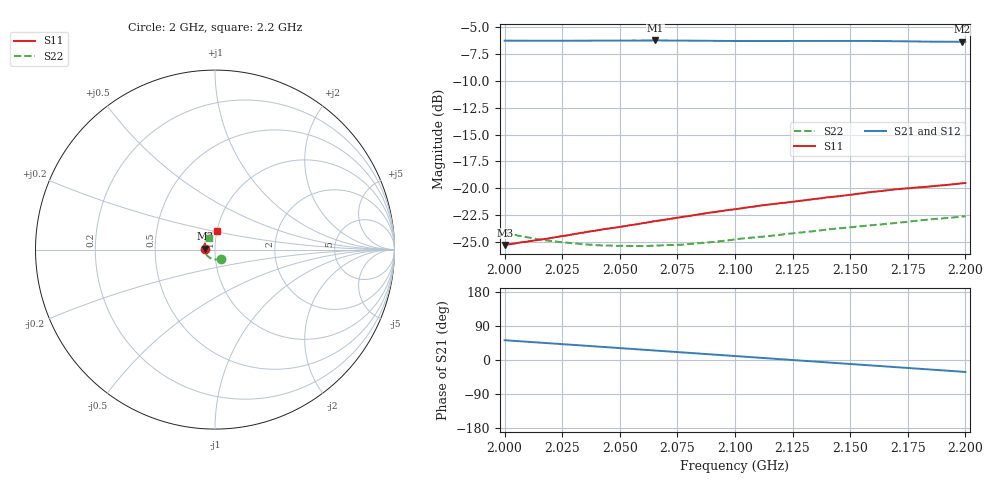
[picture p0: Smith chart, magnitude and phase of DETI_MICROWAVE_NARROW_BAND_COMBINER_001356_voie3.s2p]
! 12/28/2020 4:21:22 PM
! \\DETI-AD\SERVEUR COMMUN\0\01 - PRODUIT\0 01 356 - COMBINEUR 4 VOIES BANDE S 800 WATTS\81 -PROCES VERBAL DE CONTROLE\MESURES\07 - S2P\VOIE3.S2P
! CHANNEL.1
! TR.MEASUREMENT
! CORRECTED.DATA
# GHZ S RI R 50.0
! FREQ.GHZ  S11RE  S11IM  S21RE  S21IM  S12RE  S12IM  S22RE  S22IM
!; PortSelection: Port_12
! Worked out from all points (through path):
!   1000 points, 2 GHz to 2.2 GHz, reference 50 ohm
!   highest |S21| = -6.21 dB at 2.065 GHz (marker M1); lowest = -6.3 dB at 2.199 GHz (marker M2)
!   lowest |S11| = -25.3 dB at 2 GHz (marker M3), VSWR 1.11, Z = 44.9 + j0.549 ohm
!   |S11| at or under -10 dB: start of sweep to end of sweep
!   |S22| runs from -25.4 to -22.6 dB; largest |S21 - S12| = 0.0019
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2  -0.0541 0.00585  0.2992 0.3856  0.2991 0.3861  0.0362 -0.0502
2.0002  -0.054 0.0061  0.2998 0.385  0.2995 0.3857  0.0361 -0.0503
2.015616  -0.0556 0.0154  0.3401 0.3491  0.3405 0.3495  0.0188 -0.0544
2.024024  -0.056 0.0206  0.3609 0.3279  0.3612 0.3281  0.00939 -0.0553
2.033433  -0.0561 0.0263  0.3825 0.3027  0.3832 0.3025  -0.000761 -0.0549
2.041441  -0.0559 0.031  0.3997 0.2802  0.4002 0.28  -0.00913 -0.0534
2.048649  -0.0553 0.0353  0.4143 0.259  0.4145 0.2583  -0.0164 -0.0513
2.059459  -0.0542 0.042  0.4338 0.2251  0.4337 0.2247  -0.0266 -0.0468
2.065465  -0.0534 0.0457  0.4437 0.2058  0.4431 0.2053  -0.0319 -0.0436
2.066667  -0.0532 0.0464  0.4454 0.202  0.4449 0.2013  -0.0329 -0.043
2.077277  -0.0513 0.0527  0.4593 0.1662  0.4588 0.1659  -0.0409 -0.0361
2.091892  -0.0476 0.0613  0.4731 0.1156  0.4731 0.1157  -0.0503 -0.0253
2.1001  -0.045 0.0659  0.4785 0.0869  0.4787 0.0871  -0.0546 -0.0187
2.116517  -0.0389 0.0749  0.4851 0.0306  0.4853 0.03  -0.06 -0.00426
2.133534  -0.0311 0.0831  0.4848 -0.0292  0.4843 -0.0306  -0.062 0.0112
2.151752  -0.0213 0.0912  0.4773 -0.0946  0.4759 -0.0951  -0.0598 0.0279
2.157958  -0.0175 0.0941  0.4727 -0.1162  0.4709 -0.1163  -0.0582 0.0333
2.166767  -0.0122 0.0973  0.463 -0.1463  0.4614 -0.1459  -0.0547 0.041
2.184585  0.000433 0.1019  0.4368 -0.2055  0.4365 -0.205  -0.0459 0.0549
2.192793  0.00661 0.1037  0.4235 -0.2311  0.4236 -0.2305  -0.0407 0.0602
2.198599  0.0114 0.1048  0.4133 -0.2479  0.4133 -0.2477  -0.0369 0.064
2.2  0.0125 0.1051  0.411 -0.252  0.411 -0.252  -0.0358 0.0648
